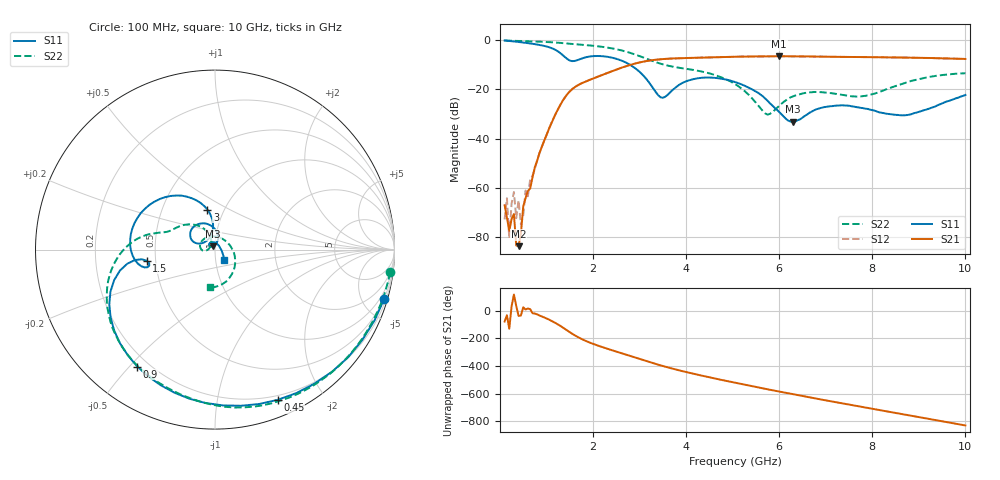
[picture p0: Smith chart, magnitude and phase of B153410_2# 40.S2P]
!  2-Port S-parameters saved by WinCal
! VAR MeasName=S-Parameters (CALIBRATED_DATA) read from VNA (N5245A)
! VAR MeasDate=2016-12-23 10:01:23
! VAR NAME=B153410_2# 40
! VAR FILENAME=B153410_2# 40.S2P
! VAR DATE=2016-12-23 10:01:23
! VAR PHYS_PORTS=1,2
# Hz S DB R 50
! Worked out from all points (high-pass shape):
!   199 points, 100 MHz to 10 GHz, reference 50 ohm
!   highest |S21| = -6.55 dB at 6 GHz (marker M1); lowest = -83.7 dB at 400 MHz (marker M2)
!   |S21| within 3 dB of the highest: 2.895 GHz to end of sweep
!   lowest |S11| = -33.2 dB at 6.3 GHz (marker M3), VSWR 1.04, Z = 48.9 + j1.86 ohm
!   |S11| at or under -10 dB: 2.793 GHz to end of sweep
!   |S22| runs from -30.3 to -0.1 dB; largest |S21 - S12| = 0.0025
!   S11 on the Smith chart (normalised r, x): 100 MHz: 0.46, -6.99; 450 MHz: 0.16, -1.49; 900 MHz: 0.16, -0.53; 1.5 GHz: 0.45, -0.06; 3 GHz: 0.83, +0.39; 10 GHz: 1.09, -0.13
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1e8  -0.16 -16.2  -67.06 -77.0  -72.83 -148.4  -0.13 -7.4
1.5e8  -0.24 -23.9  -72.13 -31.8  -64.22 55.9  -0.18 -11.0
2e8  -0.33 -31.5  -77.54 -130.1  -80.50 -109.9  -0.21 -14.3
3e8  -0.52 -46.2  -70.64 118.4  -61.70 -61.1  -0.28 -21.0
3.5e8  -0.63 -53.4  -83.43 36.0  -72.32 -17.8  -0.30 -24.3
4e8  -0.73 -60.5  -83.71 -36.4  -65.09 68.2  -0.34 -27.6
4.5e8  -0.85 -67.4  -78.64 -33.6  -74.89 18.5  -0.37 -30.9
5e8  -0.97 -74.1  -67.58 26.1  -71.45 20.9  -0.39 -34.2
5.5e8  -1.09 -80.6  -64.18 9.9  -61.09 13.2  -0.42 -37.5
9e8  -2.13 -123.6  -43.41 -40.3  -43.18 -39.3  -0.66 -60.4
1.5e9  -8.28 -170.8  -20.83 -154.3  -20.81 -154.2  -1.48 -98.2
1.75e9  -7.51 -167.3  -17.58 156.7  -17.55 157.0  -1.88 -112.6
3e9  -12.87 100.9  -9.05 11.0  -9.07 11.0  -6.49 176.0
3.4e9  -22.38 110.8  -7.86 -30.2  -7.85 -30.2  -9.27 164.4
4.15e9  -15.87 149.5  -7.18 -95.3  -7.19 -95.5  -12.09 150.7
5.05e9  -17.02 102.3  -6.75 -160.9  -6.77 -160.9  -17.84 117.3
5.75e9  -24.64 73.1  -6.57 151.2  -6.60 151.4  -30.26 151.7
6e9  -29.22 79.0  -6.55 134.9  -6.56 134.9  -26.66 -175.2
6.3e9  -33.18 119.7  -6.58 115.2  -6.60 115.3  -22.81 -177.5
6.7e9  -29.03 145.4  -6.64 89.9  -6.65 89.9  -21.16 161.1
8.35e9  -30.00 56.0  -7.00 -10.9  -7.01 -10.8  -19.60 -7.2
1e10  -22.26 -51.5  -7.65 -110.7  -7.66 -110.4  -13.45 -97.3
